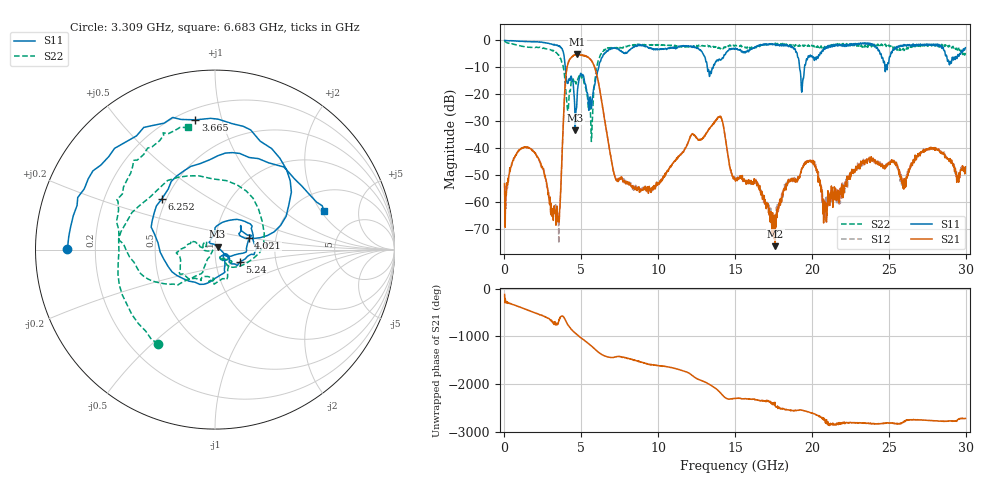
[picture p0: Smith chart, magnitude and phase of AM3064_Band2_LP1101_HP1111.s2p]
# Hz S DB R 50.0
!freq dBS11 angS11 dBS21 angS21 dBS12 angS12 dBS22 angS22
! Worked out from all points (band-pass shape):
!   1600 points, 10 MHz to 29.98 GHz, reference 50 ohm
!   highest |S21| = -5.23 dB at 4.733 GHz (marker M1); lowest = -76.4 dB at 17.61 GHz (marker M2)
!   |S21| within 3 dB of the highest: 4.158 GHz to 5.732 GHz (1.574 GHz wide, 31.8 % of centre)
!   lowest |S11| = -33.4 dB at 4.602 GHz (marker M3), VSWR 1.04, Z = 51.4 + j1.66 ohm
!   |S11| at or under -10 dB: 3.958 GHz to 6.134 GHz (2.176 GHz wide, 43.1 % of centre); 13.2 GHz to 13.57 GHz (379.1 MHz wide, 2.83 % of centre); 19.19 GHz to 19.52 GHz (323.8 MHz wide, 1.67 % of centre)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
!   |S22| runs from -37.5 to -0.3 dB; largest |S21 - S12| = 0.013
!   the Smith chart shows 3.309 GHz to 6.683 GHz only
!   S11 on the Smith chart (normalised r, x): 3.309 GHz: 0.10, +0.00; 3.665 GHz: 0.27, +0.83; 4.021 GHz: 1.45, +0.19; 5.24 GHz: 1.30, -0.19; 6.252 GHz: 0.47, +0.32; 6.683 GHz: 2.92, +2.14
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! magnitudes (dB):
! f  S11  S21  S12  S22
! 10 MHz  0.0  -53.3  -52.8  -0.3
! 1.603 GHz  -0.5  -39.8  -39.8  -2.6
! 3.309 GHz  -1.7  -64.2  -63.4  -4.3
! 3.665 GHz  -2.7  -55.5  -53.9  -6.9
! 4.021 GHz  -14.1  -11.9  -11.9  -20.6
! 4.602 GHz  -33.4  -5.4  -5.3  -15.0
! 4.733 GHz  -19.7  -5.2  -5.3  -14.5
! 5.015 GHz  -12.7  -5.5  -5.5  -14.0
! 5.24 GHz  -16.2  -5.8  -5.7  -17.0
! 5.614 GHz  -23.0  -7.2  -7.2  -30.9
! 6.252 GHz  -7.8  -20.1  -20.2  -5.3
! 6.683 GHz  -3.8  -35.4  -35.4  -3.1
! 7.283 GHz  -3.1  -51.8  -51.3  -2.7
! 10 GHz  -3.4  -53.0  -53.1  -1.8
! 13.97 GHz  -6.9  -28.5  -28.3  -2.8
! 15 GHz  -3.0  -51.7  -51.6  -1.9
! 17.61 GHz  -1.6  -76.4  -73.0  -1.1
! 19.35 GHz  -18.5  -47.6  -47.7  -2.2
! 19.99 GHz  -5.7  -44.7  -44.9  -1.8
! 20.87 GHz  -2.6  -60.0  -58.9  -2.9
! 25 GHz  -8.2  -45.4  -45.8  -1.7
! 29.98 GHz  -2.7  -46.9  -48.0  -4.6
